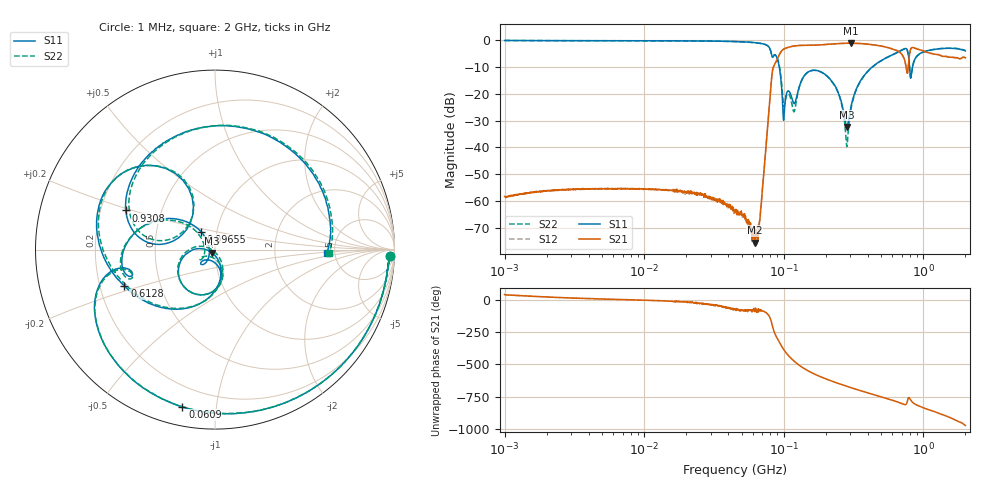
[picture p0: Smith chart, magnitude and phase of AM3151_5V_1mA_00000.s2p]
! Date/Time: Fri Jun 26 10:20:18 2020
! Network Analyzer:  Rev:
! Sweep from 1000000.0 to 2000000000.0, 1601 Points ! Power Supply: 0 V, 0 A
# HZ S DB R 50
!freq MagS11 AngS11 MagS21 AngS21 MagS12 AngS12 MagS22 AngS22
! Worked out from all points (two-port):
!   1601 points, 1 MHz to 2 GHz, reference 50 ohm
!   highest |S21| = -1.21 dB at 301.9 MHz (marker M1); lowest = -75.4 dB at 62.07 MHz (marker M2)
!   |S21| within 3 dB of the highest: 96.05 MHz to 660.4 MHz (564.4 MHz wide, 149 % of centre); 802.8 MHz to 1.016 GHz (212.8 MHz wide, 23.4 % of centre)
!   lowest |S11| = -32.4 dB at 282.5 MHz (marker M3), VSWR 1.05, Z = 48.4 - j1.79 ohm
!   |S11| at or under -10 dB: 92.81 MHz to 431.1 MHz (338.3 MHz wide, 129 % of centre); 795.8 MHz to 836.6 MHz (40.8 MHz wide, 5 % of centre)
!   |S22| runs from -39.7 to -0.2 dB; largest |S21 - S12| = 0.01
!   S11 on the Smith chart (normalised r, x): 1 MHz: 23, -39; 60.9 MHz: 0.09, -0.81; 96.55 MHz: 0.84, +0.17; 612.8 MHz: 0.31, -0.18; 930.8 MHz: 0.31, +0.19; 2 GHz: 4.32, -0.27
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1000000  -0.19 -2.2  -58.23 40.4  -58.35 38.3  -0.20 -2.1
3555161  -0.28 -5.7  -55.47 11.0  -55.56 11.0  -0.27 -5.7
1.263916e7  -0.31 -19.3  -55.55 -7.4  -55.76 -8.4  -0.31 -19.2
4.493426e7  -0.60 -70.9  -63.97 -75.7  -63.20 -67.0  -0.61 -70.9
6.090023e7  -0.96 -101.7  -72.98 -78.3  -71.95 -69.9  -0.97 -101.7
6.206852e7  -1.00 -104.2  -75.41 -79.0  -71.76 -82.3  -1.00 -104.2
6.760948e7  -1.23 -117.7  -66.24 -79.4  -66.50 -81.2  -1.25 -117.6
8.293223e7  -6.37 -165.2  -11.60 157.5  -11.60 157.5  -6.35 -163.8
9.6548e7  -17.87 128.1  -4.08 -0.1  -4.08 -0.0  -16.30 136.0
1.151013e8  -22.15 -132.7  -2.37 -102.5  -2.37 -102.6  -24.58 -141.8
1.333635e8  -15.37 -79.1  -2.02 -158.1  -2.00 -158.0  -15.42 -76.1
1.589914e8  -11.35 -113.5  -1.97 154.2  -1.96 154.2  -11.37 -113.9
2.336084e8  -17.18 -176.0  -1.45 80.7  -1.44 80.6  -17.35 178.4
2.824969e8  -32.36 -129.9  -1.24 50.2  -1.25 50.0  -39.70 -135.2
3.019241e8  -25.18 -74.2  -1.21 39.8  -1.22 39.8  -26.03 -61.0
5.652395e8  -6.16 -145.4  -2.95 -49.8  -2.94 -49.9  -6.23 -146.8
6.127825e8  -5.29 -158.1  -3.48 -61.3  -3.50 -61.2  -5.36 -159.7
7.624488e8  -3.50 140.2  -12.00 -77.4  -11.99 -77.2  -3.66 137.1
8.226611e8  -12.50 168.3  -2.94 -65.2  -2.92 -65.2  -12.44 164.1
9.30814e8  -5.30 156.3  -3.56 -102.6  -3.56 -102.7  -5.36 152.8
1.393896e9  -3.17 81.7  -6.10 -172.1  -6.09 -172.3  -3.10 78.4
2e9  -4.08 -1.7  -6.62 106.7  -6.74 106.3  -3.92 -1.8
